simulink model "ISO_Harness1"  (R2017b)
settings: Solver=FixedStepDiscrete  StartTime=0.0  StopTime=4  FixedStep=0.01  RelTol=1e-3  EnableMultiTasking=on
undefined symbols (not defined in the file): sigbuilder_block

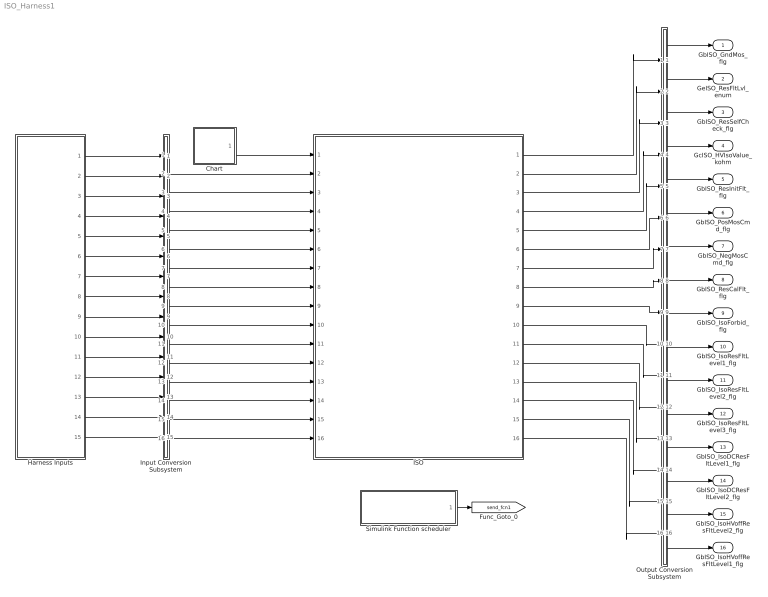
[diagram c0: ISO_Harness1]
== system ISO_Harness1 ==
  Chart : Stateflow chart  TreatAsAtomicUnit=on
  Harness Inputs : Subsystem  Tag=STV Subsys  LoadFcn=sigbuilder_block('load');  StartFcn=sigbuilder_block('start');  StopFcn=sigbuilder_block('stop');  ClipboardFcn=sigbuilder_block('clipboard');  mask(Sigbuilder block){tuvar=[0:10]}
      mask init:
      | if ~strcmp(get_param(bdroot(gcb),'SimulationStatus'),'stopped'),tuvar = sigbuilder_block('maskInit'); end
  ISO : ModelReference  ModelNameDialog=ISO  SimulationMode=Normal  ModelReferenceVersion='M114C112R114'
  Input Conversion Subsystem : Subsystem  Tag=__SLT_ICS__  Description=Signal spec. and routing
  Output Conversion Subsystem : Subsystem  Tag=__SLT_OCS__  Description=Signal spec. and routing
  Simulink Function scheduler : Test Sequence  Tag=__SLT_FCN_CALL__  TreatAsAtomicUnit=on
  GbISO_GndMos_flg : Outport  OutDataTypeStr=boolean  PortDimensions=[1]
  GeISO_ResFltLvl_enum : Outport  Port=2  OutDataTypeStr=uint8  PortDimensions=[1]
  GbISO_ResSelfCheck_flg : Outport  Port=3  OutDataTypeStr=boolean  PortDimensions=[1]
  GcISO_HVIsoValue_kohm : Outport  Port=4  OutDataTypeStr=uint16  PortDimensions=[1]
  GbISO_ResInitFlt_flg : Outport  Port=5  OutDataTypeStr=boolean  PortDimensions=[1]
  GbISO_PosMosCmd_flg : Outport  Port=6  OutDataTypeStr=boolean  PortDimensions=[1]
  GbISO_NegMosCmd_flg : Outport  Port=7  OutDataTypeStr=boolean  PortDimensions=[1]
  GbISO_ResCalFlt_flg : Outport  Port=8  OutDataTypeStr=boolean  PortDimensions=[1]
  GbISO_IsoForbid_flg : Outport  Port=9  OutDataTypeStr=boolean  PortDimensions=[1]
  GbISO_IsoResFltLevel1_flg : Outport  Port=10  OutDataTypeStr=boolean  PortDimensions=[1]
  GbISO_IsoResFltLevel2_flg : Outport  Port=11  OutDataTypeStr=boolean  PortDimensions=[1]
  GbISO_IsoResFltLevel3_flg : Outport  Port=12  OutDataTypeStr=boolean  PortDimensions=[1]
  GbISO_IsoDCResFltLevel1_flg : Outport  Port=13  OutDataTypeStr=boolean  PortDimensions=[1]
  GbISO_IsoDCResFltLevel2_flg : Outport  Port=14  OutDataTypeStr=boolean  PortDimensions=[1]
  GbISO_IsoHVoffResFltLevel2_flg : Outport  Port=15  OutDataTypeStr=boolean  PortDimensions=[1]
  GbISO_IsoHVoffResFltLevel1_flg : Outport  Port=16  OutDataTypeStr=boolean  PortDimensions=[1]
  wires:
  Harness Inputs/1(GbHDP_PackVoltVld_flg) -> Input Conversion Subsystem/1(Inport_1)
  Harness Inputs/2(GcHDP_PackVolt_V) -> Input Conversion Subsystem/2(Inport_2)
  Harness Inputs/3(GcHDP_IsoNegVolt_V) -> Input Conversion Subsystem/3(Inport_3)
  Harness Inputs/4(GbHDP_IsoNegVoltVld_flg) -> Input Conversion Subsystem/4(Inport_4)
  Harness Inputs/5(GbDCC_ChrgrISOAcv_flg) -> Input Conversion Subsystem/5(Inport_5)
  Harness Inputs/6(GeCTC_CtrCtlState_enum) -> Input Conversion Subsystem/6(Inport_6)
  Harness Inputs/7(GeMSM_BMUState_enum) -> Input Conversion Subsystem/7(Inport_7)
  Harness Inputs/8(GbNVM_ReadHVIsoValueVld_flg) -> Input Conversion Subsystem/8(Inport_8)
  Harness Inputs/9(GbUDS_MnlIsoDisable_flg) -> Input Conversion Subsystem/9(Inport_9)
  Harness Inputs/10(GbCTD_OfflineDiagFinish_flg) -> Input Conversion Subsystem/10(Inport_10)
  Harness Inputs/11(GbISP_OpenContactor_flg) -> Input Conversion Subsystem/11(Inport_11)
  Harness Inputs/12(GeCTC_CtrCtlConnMode_enum) -> Input Conversion Subsystem/12(Inport_12)
  Harness Inputs/13(GbWSM_EDCWkUpPrs_flg) -> Input Conversion Subsystem/13(Inport_13)
  Harness Inputs/14(GeLDP_CC2St_enum) -> Input Conversion Subsystem/14(Inport_14)
  Harness Inputs/15(GcISP_ShutDownHVIsoValue_kohm) -> Input Conversion Subsystem/15(Inport_15)
  Output Conversion Subsystem/1(Outport_1) -> GbISO_GndMos_flg/1
  Output Conversion Subsystem/2(Outport_2) -> GeISO_ResFltLvl_enum/1
  Output Conversion Subsystem/3(Outport_3) -> GbISO_ResSelfCheck_flg/1
  Output Conversion Subsystem/4(Outport_4) -> GcISO_HVIsoValue_kohm/1
  Output Conversion Subsystem/5(Outport_5) -> GbISO_ResInitFlt_flg/1
  Output Conversion Subsystem/6(Outport_6) -> GbISO_PosMosCmd_flg/1
  Output Conversion Subsystem/7(Outport_7) -> GbISO_NegMosCmd_flg/1
  Output Conversion Subsystem/8(Outport_8) -> GbISO_ResCalFlt_flg/1
  Output Conversion Subsystem/9(Outport_9) -> GbISO_IsoForbid_flg/1
  Output Conversion Subsystem/10(Outport_10) -> GbISO_IsoResFltLevel1_flg/1
  Output Conversion Subsystem/11(Outport_11) -> GbISO_IsoResFltLevel2_flg/1
  Output Conversion Subsystem/12(Outport_12) -> GbISO_IsoResFltLevel3_flg/1
  Output Conversion Subsystem/13(Outport_13) -> GbISO_IsoDCResFltLevel1_flg/1
  Output Conversion Subsystem/14(Outport_14) -> GbISO_IsoDCResFltLevel2_flg/1
  Output Conversion Subsystem/15(Outport_15) -> GbISO_IsoHVoffResFltLevel2_flg/1
  Output Conversion Subsystem/16(Outport_16) -> GbISO_IsoHVoffResFltLevel1_flg/1
  Input Conversion Subsystem/2(Outport_2) -> ISO/2
  Input Conversion Subsystem/3(Outport_3) -> ISO/3
  Input Conversion Subsystem/4(Outport_4) -> ISO/4
  Input Conversion Subsystem/5(Outport_5) -> ISO/5
  Input Conversion Subsystem/6(Outport_6) -> ISO/6
  Input Conversion Subsystem/7(Outport_7) -> ISO/7
  Input Conversion Subsystem/8(Outport_8) -> ISO/8
  Input Conversion Subsystem/9(Outport_9) -> ISO/9
  Input Conversion Subsystem/10(Outport_10) -> ISO/10
  Input Conversion Subsystem/11(Outport_11) -> ISO/11
  Input Conversion Subsystem/12(Outport_12) -> ISO/12
  Input Conversion Subsystem/13(Outport_13) -> ISO/13
  Input Conversion Subsystem/14(Outport_14) -> ISO/14
  Input Conversion Subsystem/15(Outport_15) -> ISO/15
  Input Conversion Subsystem/16(Outport_16) -> ISO/16
  ISO/1 -> Output Conversion Subsystem/1(Inport_1)
  ISO/2 -> Output Conversion Subsystem/2(Inport_2)
  ISO/3 -> Output Conversion Subsystem/3(Inport_3)
  ISO/4 -> Output Conversion Subsystem/4(Inport_4)
  ISO/5 -> Output Conversion Subsystem/5(Inport_5)
  ISO/6 -> Output Conversion Subsystem/6(Inport_6)
  ISO/7 -> Output Conversion Subsystem/7(Inport_7)
  ISO/8 -> Output Conversion Subsystem/8(Inport_8)
  ISO/9 -> Output Conversion Subsystem/9(Inport_9)
  ISO/10 -> Output Conversion Subsystem/10(Inport_10)
  ISO/11 -> Output Conversion Subsystem/11(Inport_11)
  ISO/12 -> Output Conversion Subsystem/12(Inport_12)
  ISO/13 -> Output Conversion Subsystem/13(Inport_13)
  ISO/14 -> Output Conversion Subsystem/14(Inport_14)
  ISO/15 -> Output Conversion Subsystem/15(Inport_15)
  ISO/16 -> Output Conversion Subsystem/16(Inport_16)
  Simulink Function scheduler/1(ISO_Insulation_100ms()) -> [send_fcn1]
  Chart/1(Run10ms()) -> ISO/1

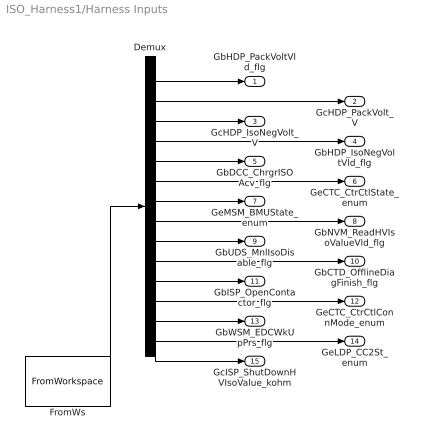
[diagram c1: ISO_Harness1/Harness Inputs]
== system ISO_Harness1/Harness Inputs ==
  Demux : Demux  Tag=STV Demux  Outputs=15
  FromWs : FromWorkspace  Tag=STV FromWs  VariableName=tuvar  SampleTime=0
  GbHDP_PackVoltVld_flg : Outport  Tag=STV Outport
  GcHDP_PackVolt_V : Outport  Tag=STV Outport  Port=2
  GcHDP_IsoNegVolt_V : Outport  Tag=STV Outport  Port=3
  GbHDP_IsoNegVoltVld_flg : Outport  Tag=STV Outport  Port=4
  GbDCC_ChrgrISOAcv_flg : Outport  Tag=STV Outport  Port=5
  GeCTC_CtrCtlState_enum : Outport  Tag=STV Outport  Port=6
  GeMSM_BMUState_enum : Outport  Tag=STV Outport  Port=7
  GbNVM_ReadHVIsoValueVld_flg : Outport  Tag=STV Outport  Port=8
  GbUDS_MnlIsoDisable_flg : Outport  Tag=STV Outport  Port=9
  GbCTD_OfflineDiagFinish_flg : Outport  Tag=STV Outport  Port=10
  GbISP_OpenContactor_flg : Outport  Tag=STV Outport  Port=11
  GeCTC_CtrCtlConnMode_enum : Outport  Tag=STV Outport  Port=12
  GbWSM_EDCWkUpPrs_flg : Outport  Tag=STV Outport  Port=13
  GeLDP_CC2St_enum : Outport  Tag=STV Outport  Port=14
  GcISP_ShutDownHVIsoValue_kohm : Outport  Tag=STV Outport  Port=15
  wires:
  FromWs/1 -> Demux/1
  Demux/1 -> GbHDP_PackVoltVld_flg/1
  Demux/2 -> GcHDP_PackVolt_V/1
  Demux/3 -> GcHDP_IsoNegVolt_V/1
  Demux/4 -> GbHDP_IsoNegVoltVld_flg/1
  Demux/5 -> GbDCC_ChrgrISOAcv_flg/1
  Demux/6 -> GeCTC_CtrCtlState_enum/1
  Demux/7 -> GeMSM_BMUState_enum/1
  Demux/8 -> GbNVM_ReadHVIsoValueVld_flg/1
  Demux/9 -> GbUDS_MnlIsoDisable_flg/1
  Demux/10 -> GbCTD_OfflineDiagFinish_flg/1
  Demux/11 -> GbISP_OpenContactor_flg/1
  Demux/12 -> GeCTC_CtrCtlConnMode_enum/1
  Demux/13 -> GbWSM_EDCWkUpPrs_flg/1
  Demux/14 -> GeLDP_CC2St_enum/1
  Demux/15 -> GcISP_ShutDownHVIsoValue_kohm/1

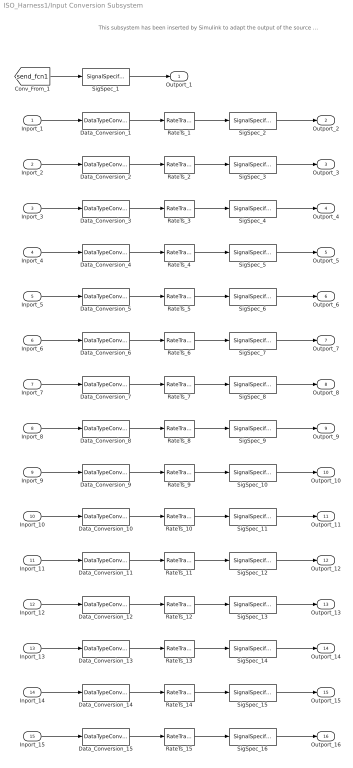
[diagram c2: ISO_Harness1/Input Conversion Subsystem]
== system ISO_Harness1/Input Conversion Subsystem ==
  note: This subsystem has been inserted by Simulink to adapt the output of the source blocks to the interface required by the harnessed component. Modifying the contents of this subsystem may result in compilation and simulation failure.
  Inport_1 : Inport
  Inport_2 : Inport  Port=2
  Inport_3 : Inport  Port=3
  Inport_4 : Inport  Port=4
  Inport_5 : Inport  Port=5
  Inport_6 : Inport  Port=6
  Inport_7 : Inport  Port=7
  Inport_8 : Inport  Port=8
  Inport_9 : Inport  Port=9
  Inport_10 : Inport  Port=10
  Inport_11 : Inport  Port=11
  Inport_12 : Inport  Port=12
  Inport_13 : Inport  Port=13
  Inport_14 : Inport  Port=14
  Inport_15 : Inport  Port=15
  Data_Conversion_{1,4..5,8..11,13} (8 alike) : DataTypeConversion  OutDataTypeStr=boolean
  Data_Conversion_{6..7,12,14} (4 alike) : DataTypeConversion  OutDataTypeStr=uint8
  Data_Conversion_15 : DataTypeConversion  OutDataTypeStr=uint16
  Data_Conversion_2 : DataTypeConversion  OutDataTypeStr=single
  Data_Conversion_3 : DataTypeConversion  OutDataTypeStr=single
  RateTs_{1..15} (15 alike) : RateTransition
  SigSpec_1 : SignalSpecification
  SigSpec_{2,6,9..12} (6 alike) : SignalSpecification  OutDataTypeStr=boolean  Unit=flag  Dimensions=[1]
  SigSpec_{7..8,13,15} (4 alike) : SignalSpecification  OutDataTypeStr=uint8  Unit=enum  Dimensions=[1]
  SigSpec_14 : SignalSpecification  OutDataTypeStr=boolean  Unit=flg  Dimensions=[1]
  SigSpec_16 : SignalSpecification  OutDataTypeStr=uint16  Unit=kohm  Dimensions=[1]
  SigSpec_3 : SignalSpecification  OutDataTypeStr=single  Unit=V  Dimensions=[1]
  SigSpec_4 : SignalSpecification  OutDataTypeStr=single  Unit=V  Dimensions=[1]
  SigSpec_5 : SignalSpecification  OutDataTypeStr=boolean  Unit=flg  Dimensions=[1]
  Outport_1 : Outport
  Outport_2 : Outport  Port=2
  Outport_3 : Outport  Port=3
  Outport_4 : Outport  Port=4
  Outport_5 : Outport  Port=5
  Outport_6 : Outport  Port=6
  Outport_7 : Outport  Port=7
  Outport_8 : Outport  Port=8
  Outport_9 : Outport  Port=9
  Outport_10 : Outport  Port=10
  Outport_11 : Outport  Port=11
  Outport_12 : Outport  Port=12
  Outport_13 : Outport  Port=13
  Outport_14 : Outport  Port=14
  Outport_15 : Outport  Port=15
  Outport_16 : Outport  Port=16
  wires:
  SigSpec_1/1 -> Outport_1/1
  [send_fcn1] -> SigSpec_1/1
  SigSpec_2/1 -> Outport_2/1
  RateTs_1/1 -> SigSpec_2/1
  Data_Conversion_1/1 -> RateTs_1/1
  Inport_1/1 -> Data_Conversion_1/1
  SigSpec_3/1 -> Outport_3/1
  RateTs_2/1 -> SigSpec_3/1
  Data_Conversion_2/1 -> RateTs_2/1
  Inport_2/1 -> Data_Conversion_2/1
  SigSpec_4/1 -> Outport_4/1
  RateTs_3/1 -> SigSpec_4/1
  Data_Conversion_3/1 -> RateTs_3/1
  Inport_3/1 -> Data_Conversion_3/1
  SigSpec_5/1 -> Outport_5/1
  RateTs_4/1 -> SigSpec_5/1
  Data_Conversion_4/1 -> RateTs_4/1
  Inport_4/1 -> Data_Conversion_4/1
  SigSpec_6/1 -> Outport_6/1
  RateTs_5/1 -> SigSpec_6/1
  Data_Conversion_5/1 -> RateTs_5/1
  Inport_5/1 -> Data_Conversion_5/1
  SigSpec_7/1 -> Outport_7/1
  RateTs_6/1 -> SigSpec_7/1
  Data_Conversion_6/1 -> RateTs_6/1
  Inport_6/1 -> Data_Conversion_6/1
  SigSpec_8/1 -> Outport_8/1
  RateTs_7/1 -> SigSpec_8/1
  Data_Conversion_7/1 -> RateTs_7/1
  Inport_7/1 -> Data_Conversion_7/1
  SigSpec_9/1 -> Outport_9/1
  RateTs_8/1 -> SigSpec_9/1
  Data_Conversion_8/1 -> RateTs_8/1
  Inport_8/1 -> Data_Conversion_8/1
  SigSpec_10/1 -> Outport_10/1
  RateTs_9/1 -> SigSpec_10/1
  Data_Conversion_9/1 -> RateTs_9/1
  Inport_9/1 -> Data_Conversion_9/1
  SigSpec_11/1 -> Outport_11/1
  RateTs_10/1 -> SigSpec_11/1
  Data_Conversion_10/1 -> RateTs_10/1
  Inport_10/1 -> Data_Conversion_10/1
  SigSpec_12/1 -> Outport_12/1
  RateTs_11/1 -> SigSpec_12/1
  Data_Conversion_11/1 -> RateTs_11/1
  Inport_11/1 -> Data_Conversion_11/1
  SigSpec_13/1 -> Outport_13/1
  RateTs_12/1 -> SigSpec_13/1
  Data_Conversion_12/1 -> RateTs_12/1
  Inport_12/1 -> Data_Conversion_12/1
  SigSpec_14/1 -> Outport_14/1
  RateTs_13/1 -> SigSpec_14/1
  Data_Conversion_13/1 -> RateTs_13/1
  Inport_13/1 -> Data_Conversion_13/1
  SigSpec_15/1 -> Outport_15/1
  RateTs_14/1 -> SigSpec_15/1
  Data_Conversion_14/1 -> RateTs_14/1
  Inport_14/1 -> Data_Conversion_14/1
  SigSpec_16/1 -> Outport_16/1
  RateTs_15/1 -> SigSpec_16/1
  Data_Conversion_15/1 -> RateTs_15/1
  Inport_15/1 -> Data_Conversion_15/1

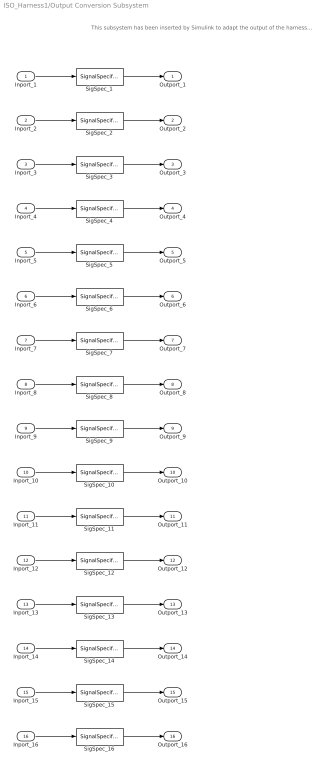
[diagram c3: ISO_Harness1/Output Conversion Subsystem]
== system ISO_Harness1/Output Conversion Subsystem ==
  note: This subsystem has been inserted by Simulink to adapt the output of the harnessed component to the interface required by the sink blocks. Modifying the contents of this subsystem may result in compilation and simulation failure.
  Inport_1 : Inport
  Inport_2 : Inport  Port=2
  Inport_3 : Inport  Port=3
  Inport_4 : Inport  Port=4
  Inport_5 : Inport  Port=5
  Inport_6 : Inport  Port=6
  Inport_7 : Inport  Port=7
  Inport_8 : Inport  Port=8
  Inport_9 : Inport  Port=9
  Inport_10 : Inport  Port=10
  Inport_11 : Inport  Port=11
  Inport_12 : Inport  Port=12
  Inport_13 : Inport  Port=13
  Inport_14 : Inport  Port=14
  Inport_15 : Inport  Port=15
  Inport_16 : Inport  Port=16
  SigSpec_{1,3,5..16} (14 alike) : SignalSpecification  OutDataTypeStr=boolean  Unit=flag  Dimensions=[1]
  SigSpec_2 : SignalSpecification  OutDataTypeStr=uint8  Unit=enum  Dimensions=[1]
  SigSpec_4 : SignalSpecification  OutDataTypeStr=uint16  Unit=kohm  Dimensions=[1]
  Outport_1 : Outport
  Outport_2 : Outport  Port=2
  Outport_3 : Outport  Port=3
  Outport_4 : Outport  Port=4
  Outport_5 : Outport  Port=5
  Outport_6 : Outport  Port=6
  Outport_7 : Outport  Port=7
  Outport_8 : Outport  Port=8
  Outport_9 : Outport  Port=9
  Outport_10 : Outport  Port=10
  Outport_11 : Outport  Port=11
  Outport_12 : Outport  Port=12
  Outport_13 : Outport  Port=13
  Outport_14 : Outport  Port=14
  Outport_15 : Outport  Port=15
  Outport_16 : Outport  Port=16
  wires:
  Inport_1/1 -> SigSpec_1/1
  SigSpec_1/1 -> Outport_1/1
  Inport_2/1 -> SigSpec_2/1
  SigSpec_2/1 -> Outport_2/1
  Inport_3/1 -> SigSpec_3/1
  SigSpec_3/1 -> Outport_3/1
  Inport_4/1 -> SigSpec_4/1
  SigSpec_4/1 -> Outport_4/1
  Inport_5/1 -> SigSpec_5/1
  SigSpec_5/1 -> Outport_5/1
  Inport_6/1 -> SigSpec_6/1
  SigSpec_6/1 -> Outport_6/1
  Inport_7/1 -> SigSpec_7/1
  SigSpec_7/1 -> Outport_7/1
  Inport_8/1 -> SigSpec_8/1
  SigSpec_8/1 -> Outport_8/1
  Inport_9/1 -> SigSpec_9/1
  SigSpec_9/1 -> Outport_9/1
  Inport_10/1 -> SigSpec_10/1
  SigSpec_10/1 -> Outport_10/1
  Inport_11/1 -> SigSpec_11/1
  SigSpec_11/1 -> Outport_11/1
  Inport_12/1 -> SigSpec_12/1
  SigSpec_12/1 -> Outport_12/1
  Inport_13/1 -> SigSpec_13/1
  SigSpec_13/1 -> Outport_13/1
  Inport_14/1 -> SigSpec_14/1
  SigSpec_14/1 -> Outport_14/1
  Inport_15/1 -> SigSpec_15/1
  SigSpec_15/1 -> Outport_15/1
  Inport_16/1 -> SigSpec_16/1
  SigSpec_16/1 -> Outport_16/1

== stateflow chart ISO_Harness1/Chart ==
  (default) -> (junction 1)
  (junction 1) -> (junction 3) : {Run10ms}
  events: output FUNCTION_CALL_EVENT

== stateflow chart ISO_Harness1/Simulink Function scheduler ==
  state Run
  state AsyncFunctionCalls
    % Call Asynchronous FunctionCall Subsystems.
    %
    %% Schedule function-call outputs.
    %% Modify this code to change function-call order.
    send(ISO_Insulation_100ms)
  (default) -> Run
  events: output FUNCTION_CALL_EVENT
